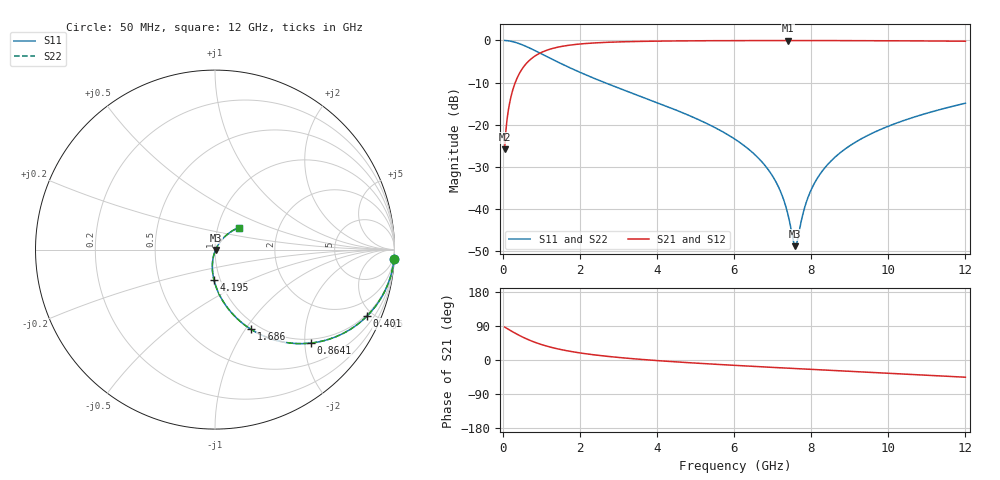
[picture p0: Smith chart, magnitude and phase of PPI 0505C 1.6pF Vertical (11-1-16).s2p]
# GHz S MA R 50
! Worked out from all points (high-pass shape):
!   1601 points, 50 MHz to 12 GHz, reference 50 ohm
!   highest |S21| = -0.04 dB at 7.392 GHz (marker M1); lowest = -25.9 dB at 50 MHz (marker M2)
!   |S21| within 3 dB of the highest: 964.5 MHz to end of sweep
!   lowest |S11| = -48.9 dB at 7.586 GHz (marker M3), VSWR 1.01, Z = 50.3 - j0.155 ohm
!   |S11| at or under -10 dB: 2.639 GHz to end of sweep
!   |S22| runs from -48.9 to 0.0 dB; largest |S21 - S12| = 0
!   S11 on the Smith chart (normalised r, x): 50 MHz: 1, -37; 401 MHz: 0.91, -4.64; 864.1 MHz: 0.91, -2.14; 1.686 GHz: 0.91, -1.06; 4.195 GHz: 0.93, -0.32; 12 GHz: 1.26, +0.32
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0.05  0.9987 -3.1  0.0509 86.9  0.0509 86.9  0.9987 -3.1
0.199375  0.9799 -12.1  0.1992 77.9  0.1992 77.9  0.9799 -12.1
0.4010313  0.9251 -23.5  0.379 66.5  0.379 66.5  0.9251 -23.5
0.8640937  0.7463 -44.2  0.6643 45.7  0.6643 45.7  0.7463 -44.2
1.252469  0.6073 -56.2  0.7929 33.6  0.7929 33.6  0.6073 -56.2
1.685656  0.4867 -65.8  0.8716 24.0  0.8716 24.0  0.4867 -65.8
2.044156  0.4105 -71.7  0.9098 18.1  0.9098 18.1  0.4105 -71.7
4.038312  0.1799 -90.9  0.9808 -1.8  0.9808 -1.8  0.1799 -90.9
4.195156  0.1687 -92.0  0.9827 -2.9  0.9827 -2.9  0.1687 -92.0
6.025  0.06705 -101.5  0.9942 -14.2  0.9942 -14.2  0.06705 -101.5
6.913781  0.02804 -102.0  0.9958 -19.0  0.9958 -19.0  0.02804 -102.0
7.190125  0.01668 -98.4  0.9959 -20.5  0.9959 -20.5  0.01668 -98.4
7.391781  0.00879 -87.8  0.996 -21.6  0.996 -21.6  0.00879 -87.8
7.533688  0.004245 -54.8  0.9959 -22.3  0.9959 -22.3  0.004245 -54.8
7.585969  0.003597 -25.3  0.9959 -22.6  0.9959 -22.6  0.003597 -25.3
7.645719  0.004247 8.9  0.9959 -22.9  0.9959 -22.9  0.004247 8.9
7.847375  0.01095 46.5  0.9958 -23.9  0.9958 -23.9  0.01095 46.5
8.019156  0.01756 53.0  0.9956 -24.8  0.9956 -24.8  0.01756 53.0
8.325375  0.02953 56.2  0.9952 -26.4  0.9952 -26.4  0.02953 56.2
8.743625  0.04592 56.6  0.9945 -28.5  0.9945 -28.5  0.04592 56.6
10.01331  0.09615 52.4  0.9904 -35.0  0.9904 -35.0  0.09615 52.4
12  0.1794 43.0  0.9781 -45.4  0.9781 -45.4  0.1794 43.0
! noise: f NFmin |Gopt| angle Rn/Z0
0.05  0.0009255  0.956  1.698  0.004739
1.372  0.005214  0.7434  5.934  0.004067
2.701  0.00808  0.6835  9.519  0.004916
4.031  0.01059  0.6478  13.14  0.005633
5.36  0.01295  0.6236  16.73  0.006301
6.682  0.01522  0.6071  20.23  0.00696
8.012  0.01751  0.5959  23.68  0.007648
9.341  0.01984  0.5892  27.05  0.008386
10.67  0.02227  0.5862  30.34  0.009199
12  0.02482  0.5866  33.55  0.01011
